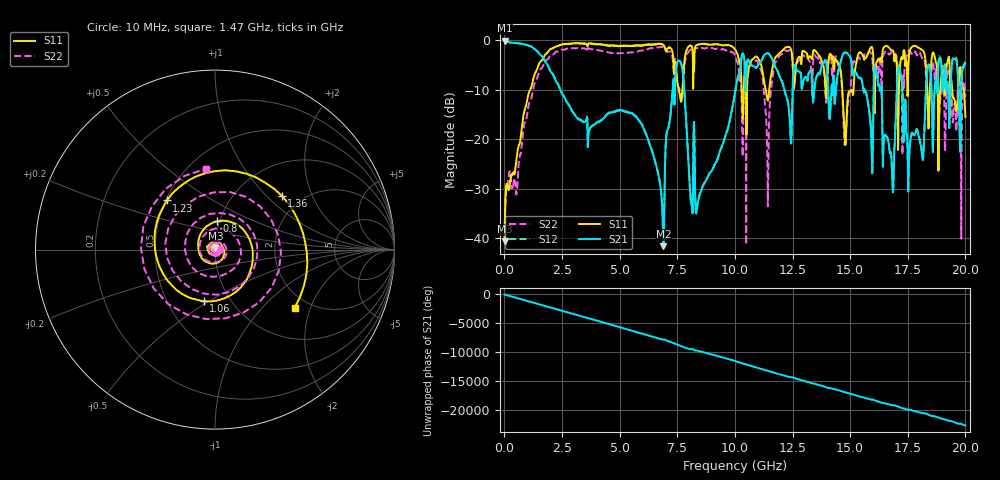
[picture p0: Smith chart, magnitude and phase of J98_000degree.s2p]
!Keysight Technologies,N5222A,MY51421036,A.10.65.16
!Date: Friday, March 31, 2023 14:37:21
!Correction: S11(Full 2 Port(1,2))
!S21(Full 2 Port(1,2))
!S12(Full 2 Port(1,2))
!S22(Full 2 Port(1,2))
!S2P File: Measurements: S11, S21, S12, S22:
# Hz S  dB  R 50
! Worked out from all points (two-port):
!   2000 points, 10 MHz to 20 GHz, reference 50 ohm
!   highest |S21| = -0.06 dB at 10 MHz (marker M1); lowest = -41.6 dB at 6.9 GHz (marker M2)
!   |S21| within 3 dB of the highest: start of sweep to 1.589 GHz; 14.67 GHz to 14.95 GHz (286.9 MHz wide, 1.94 % of centre)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
!   lowest |S11| = -40.6 dB at 10 MHz (marker M3), VSWR 1.02, Z = 50.2 + j0.909 ohm
!   |S11| at or under -10 dB: start of sweep to 1.118 GHz; 14.66 GHz to 15.15 GHz (484.7 MHz wide, 3.25 % of centre); 19.42 GHz to 19.69 GHz (267.9 MHz wide, 1.37 % of centre)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
!   |S22| runs from -41.2 to -1.3 dB; largest |S21 - S12| = 0.04
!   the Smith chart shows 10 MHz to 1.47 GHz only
!   S11 on the Smith chart (normalised r, x): 10 MHz: 1.00, +0.02; 800 MHz: 0.98, +0.32; 1.06 GHz: 0.75, -0.47; 1.23 GHz: 0.51, +0.33; 1.36 GHz: 1.59, +1.24; 1.47 GHz: 1.68, -1.57
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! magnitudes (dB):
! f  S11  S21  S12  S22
! 10 MHz  -40.6  -0.1  0.0  -39.7
! 800 MHz  -16.0  -0.8  -0.7  -18.9
! 1.06 GHz  -10.6  -1.1  -1.1  -12.9
! 1.23 GHz  -8.3  -1.5  -1.4  -10.5
! 1.36 GHz  -6.4  -2.0  -1.9  -8.2
! 1.47 GHz  -5.2  -2.5  -2.4  -6.9
! 3.35 GHz  -0.6  -16.3  -16.2  -1.7
! 6.68 GHz  -0.8  -27.1  -27.0  -1.5
! 6.9 GHz  -1.0  -41.6  -41.5  -1.4
! 7.55 GHz  -9.6  -4.1  -4.0  -9.4
! 8.38 GHz  -0.9  -33.1  -33.1  -1.6
! 10.01 GHz  -1.9  -10.5  -10.4  -3.0
! 11.41 GHz  -12.0  -2.6  -2.6  -24.5
! 11.88 GHz  -2.9  -6.6  -6.6  -3.7
! 13.34 GHz  -3.8  -6.8  -6.8  -9.7
! 14.44 GHz  -4.3  -7.5  -7.4  -4.0
! 14.79 GHz  -21.1  -2.5  -2.4  -20.6
! 16.67 GHz  -1.4  -20.7  -20.6  -2.7
! 17.14 GHz  -6.7  -5.5  -5.4  -7.2
! 17.56 GHz  -2.7  -23.7  -23.5  -2.1
! 18.4 GHz  -17.8  -5.1  -4.9  -11.8
! 20 GHz  -15.5  -4.8  -4.3  -11.4
